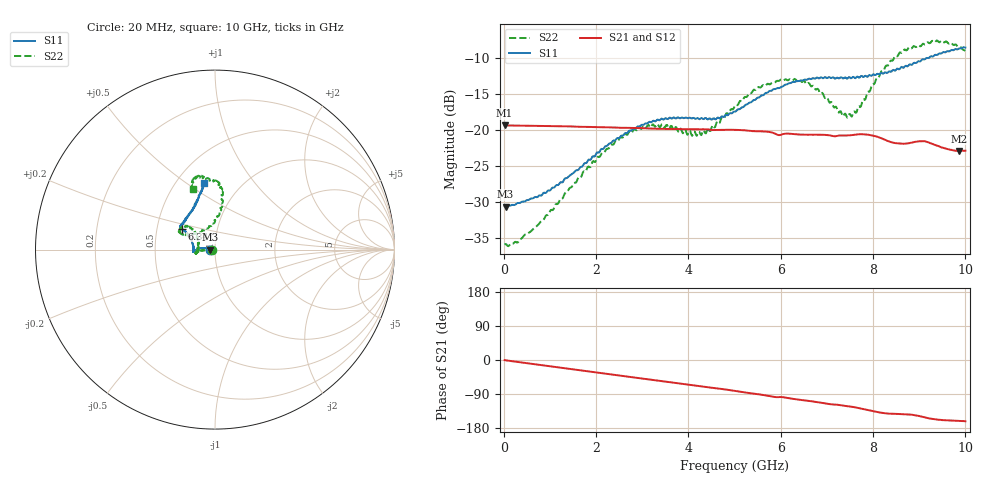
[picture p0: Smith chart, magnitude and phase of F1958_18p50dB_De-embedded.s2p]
! Integrated Device Technology
! Corporate Headquarters
! 6024 Silver Creek Valley Road
! San Jose, CA 95138  USA
! Phone:  1-408-284-8200
! Toll Free:  1-800-223-1366
! Webpage:  http://www.idt.com/
! Timing and RF Division
! 515 Groton Road, Suite 102
! Westford, MA 01886-6024
! Device:  F1958
! Description: 7-bit 0.25 dB Digital Step Attenuator
! Frequency:  0.001 -  6.000 GHz
! Package:  4x4 mm Thin QFN Plastic Package: 24 pin
! Ports:  2 RF, 12 DC
!  Pin  1  = D0
!  Pin  2  = VDD
!  Pin  3  = VMODE
!  Pin  4  = GND
!  Pin  5  = RF1  =  Port 1
!  Pin  6  = GND
!  Pin  7  = GND
!  Pin  8  = GND
!  Pin  9  = GND
!  Pin 10  = GND
!  Pin 11  = GND
!  Pin 12  = GND
!  Pin 13  = GND
!  Pin 14  = RF2  =  Port 2
!  Pin 15  = GND
!  Pin 16  = LE
!  Pin 17  = CLK
!  Pin 18  = DATA
!  Pin 19  = D6
!  Pin 20  = D5
!  Pin 21  = D4
!  Pin 22  = D3
!  Pin 23  = D2
!  Pin 24  = D1
! State:  74
! Atten State:  18.50 dB
! Voltage:  +3.30 Volts
! Current:  0.258 mA
! Data:  The device was measured on a F1958 evaluation board which has
!  individual transmission lines to the RF pins.  Data was collected
!  using a calibrated network analyzer.  The evaluation board was
!  de-embedded using Automatic Fixture Removal (AFR).
!  The reference plane is the edge of the package pin.
! Misc:
!  Action Tracker AT0419
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# GHz S dB R 50
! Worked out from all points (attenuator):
!   500 points, 20 MHz to 10 GHz, reference 50 ohm
!   highest |S21| = -19.31 dB at 20 MHz (marker M1); lowest = -22.9 dB at 9.86 GHz (marker M2)
!   lowest |S11| = -30.6 dB at 40 MHz (marker M3), VSWR 1.06, Z = 47.1 - j0.0454 ohm
!   |S11| at or under -10 dB: start of sweep to 9.143 GHz
!   |S22| runs from -36.1 to -7.5 dB; largest |S21 - S12| = 0.00036
!   S11 on the Smith chart (normalised r, x): 20 MHz: 0.94, -0.00; 6.34 GHz: 0.67, +0.16; 10 GHz: 0.68, +0.58
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0.02  -30.59 -178.8  -19.31 -0.4  -19.31 -0.4  -35.93 -177.1
0.04  -30.61 -179.1  -19.32 -0.7  -19.32 -0.7  -35.83 -175.7
0.32  -30.12 175.3  -19.35 -5.4  -19.35 -5.4  -35.50 -179.1
0.72  -29.32 173.1  -19.38 -12.0  -19.38 -12.0  -33.31 -176.2
1.7  -25.06 172.1  -19.51 -27.9  -19.50 -27.9  -26.12 -177.5
2.6  -20.64 178.0  -19.65 -42.4  -19.63 -42.5  -20.78 -174.5
2.92  -19.48 -178.3  -19.69 -47.7  -19.68 -47.8  -19.57 -171.6
3.36  -18.59 -174.8  -19.79 -54.9  -19.78 -55.0  -19.42 -167.6
4.24  -18.46 -178.3  -19.86 -68.9  -19.87 -68.9  -20.23 169.7
4.5  -18.53 175.9  -19.95 -73.5  -19.96 -73.5  -19.68 153.5
5.02  -17.39 161.4  -19.94 -81.7  -19.95 -81.7  -16.47 139.2
5.56  -15.27 150.9  -20.15 -91.1  -20.16 -91.1  -14.06 139.9
6.34  -13.16 147.9  -20.55 -103.8  -20.57 -103.8  -13.08 153.4
6.68  -12.79 146.7  -20.61 -109.1  -20.63 -109.0  -13.85 153.7
7.3  -12.61 140.9  -20.73 -119.4  -20.73 -119.3  -17.34 132.4
7.5  -12.64 138.2  -20.70 -122.8  -20.70 -122.7  -17.72 113.5
7.68  -12.60 135.3  -20.56 -126.5  -20.56 -126.5  -16.71 96.1
8.34  -11.81 119.1  -21.54 -141.5  -21.54 -141.6  -10.82 81.2
8.68  -11.16 112.4  -21.86 -143.1  -21.88 -143.1  -8.75 86.0
9.26  -9.68 104.7  -21.84 -155.1  -21.86 -155.2  -7.67 99.3
9.86  -8.62 99.8  -22.89 -160.3  -22.90 -160.3  -8.41 108.9
10  -8.48 99.7  -22.83 -161.5  -22.85 -161.4  -8.95 109.9
